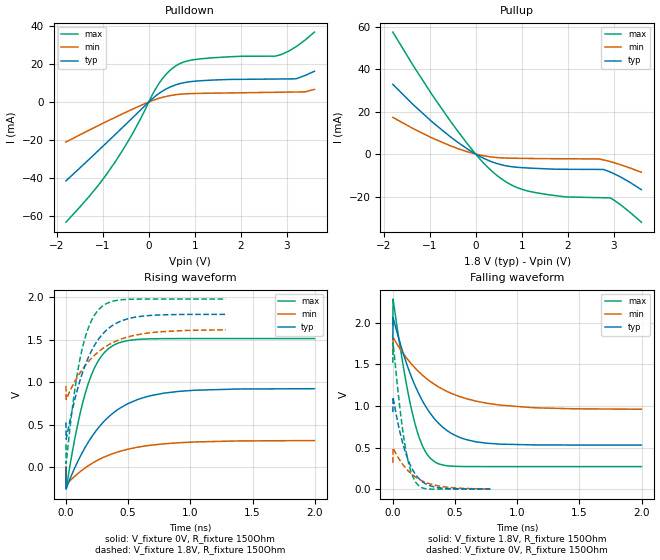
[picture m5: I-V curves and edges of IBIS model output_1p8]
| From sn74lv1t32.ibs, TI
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|   output_1p8 Model
[Model]   output_1p8
Model_type   Output
Polarity   Inverting
Vmeas = 0.9
Vref = 0
Cref = 30pF
Rref = 500
|   typ   min   max
|   (nom PVT)   (fast PVT)   (slow PVT)
C_comp   1.625e-12   1.538e-12   1.747e-12
| Where nom  PVT is Nominal Process, 1.8V, 40C
|   Fast PVT is Strong Process,  1.98V, -40C
|   Slow PVT is Weak Process,   1.62V, 140C
[Voltage Range]   1.8   1.62   1.98
|Junction Temperature
[Temperature Range]   40   140   -40
[Pullup Reference]   1.8   1.62   1.98
[Pulldown Reference]   0   0   0
[Power Clamp Reference]   1.8   1.62   1.98
[GND Clamp Reference]   0   0   0
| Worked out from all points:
|   slope of the pulldown table from 0 to 0.27 V, typ, clamps not added: 51.4 ohm
|   slope of the pullup table from 0 to 0.27 V, typ, clamps not added: 91.8 ohm
|   falling waveform, V_fixture 1.8V, R_fixture 150Ohm: 20-80 % time 271ps typ, 422ps min, 147ps max; typ from 1.8 V to 0.529 V
|   rising waveform, V_fixture 0V, R_fixture 150Ohm: 20-80 % time 351ps typ, 413ps min, 178ps max; typ from 0 V to 0.926 V
|   rising waveform, V_fixture 1.8V, R_fixture 150Ohm: 20-80 % time 213ps typ, 300ps min, 135ps max; typ from 0.529 V to 1.8 V
|   falling waveform, V_fixture 0V, R_fixture 150Ohm: 20-80 % time 129ps typ, 192ps min, 89.2ps max; typ from 0.926 V to 0.001 V
[Pulldown]
|   Voltage   I(typ)   I(min)   I(max)
-1.8V     -41.38mA   -20.97mA   -63.01mA
-1.282V   -29.71mA   -14.59mA   -49.12mA
-907.4mV  -21.14mA   -10.11mA   -37.57mA
-346.7mV  -8.144mA   -3.699mA   -16.34mA
146.3mV   3.113mA    1.347mA    6.829mA
308.7mV   5.851mA    2.524mA    12.6mA
496.8mV   8.174mA    3.493mA    17.32mA
684.9mV   9.69mA     4.077mA    20.23mA
996.1mV   10.89mA    4.456mA    22.24mA
2.832V    12.05mA    5.11mA     24.55mA
3.196V    12.13mA    5.233mA    28.93mA
3.6V      16.12mA    6.605mA    36.64mA
[Pullup]
|   Voltage   I(typ)   I(min)   I(max)
-1.8V     32.8mA     17.27mA    57.44mA
-964.4mV  15.51mA    7.761mA    28.52mA
-368.5mV  5.222mA    2.43mA     10.19mA
79.2mV    -961.8uA   -401.8uA   -2.013mA
528.5mV   -4.873mA   -1.755mA   -11.17mA
898.9mV   -6.226mA   -2.004mA   -15.78mA
1.331V    -6.775mA   -2.129mA   -18.29mA
1.978V    -7.178mA   -2.225mA   -20.21mA
2.776V    -7.258mA   -2.752mA   -20.58mA
2.926V    -8.494mA   -3.575mA   -20.65mA
3.17V     -11.06mA   -5.172mA   -24.25mA
3.6V      -16.77mA   -8.595mA   -32.09mA
[Ramp]
R_load = 150
|   typ   min   max
dV/dt_r   0.55539/3.51261e-10   0.189425/4.12478e-10   0.909405/1.77611e-10
dV/dt_f   0.762438/2.70787e-10   0.396415/4.2157e-10   1.02562/1.47306e-10
[Falling Waveform]
V_fixture = 1.8V
V_fixture_min = 1.62V
V_fixture_max = 1.98V
R_fixture = 150Ohm
|   Time   V(typ)   V(min)   V(max)
0s        1.8V       1.62V      1.98V
2ps       2.062V     1.822V     2.282V
110ps     1.51V      1.576V     1.255V
156ps     1.324V     1.492V     919.1mV
198ps     1.179V     1.425V     682.8mV
264ps     993.6mV    1.336V     445.1mV
344ps     828.8mV    1.249V     321.2mV
522ps     630.9mV    1.12V      273.1mV
754ps     551.8mV    1.032V     270.8mV
1.998ns   529.3mV    959.3mV    270.6mV
[Rising Waveform]
V_fixture = 0V
V_fixture_min = 0V
V_fixture_max = 0V
R_fixture = 150Ohm
|   Time   V(typ)   V(min)   V(max)
0s        377.5pV    9.214nV    426.7pV
2ps       -247.9mV   -204.4mV   -256.3mV
52ps      -67.54mV   -130.2mV   187.9mV
104ps     96.47mV    -62.83mV   570.1mV
204ps     352.7mV    41.84mV    1.084V
288ps     512.7mV    108.5mV    1.314V
388ps     649.1mV    167.6mV    1.441V
610ps     814.4mV    245.6mV    1.508V
902ps     893.2mV    289.4mV    1.515V
1.998ns   925.6mV    315.7mV    1.516V
[Rising Waveform]
V_fixture = 1.8V
V_fixture_min = 1.62V
V_fixture_max = 1.98V
R_fixture = 150Ohm
|   Time   V(typ)   V(min)   V(max)
0s        529.2mV    958.3mV    270.6mV
2ps       331.6mV    800.7mV    44.91mV
42ps      615.2mV    928mV      584.8mV
72ps      803mV      1.012V     921.9mV
138ps     1.135V     1.165V     1.439V
204ps     1.367V     1.282V     1.722V
290ps     1.56V      1.392V     1.893V
394ps     1.687V     1.48V      1.961V
562ps     1.769V     1.557V     1.979V
1.286ns   1.8V       1.618V     1.98V
[Falling Waveform]
V_fixture = 0V
V_fixture_min = 0V
V_fixture_max = 0V
R_fixture = 150Ohm
|   Time   V(typ)   V(min)   V(max)
0s        926mV      316.5mV    1.516V
2ps       1.104V     493.9mV    1.76V
52ps      719.6mV    357.6mV    1.037V
74ps      583.8mV    308.7mV    769.3mV
98ps      458.1mV    262.3mV    527.3mV
138ps     297mV      198.8mV    247.4mV
192ps     157.3mV    135.6mV    66.82mV
258ps     69.23mV    84.64mV    6.244mV
350ps     21.68mV    43.64mV    155.8uV
784ps     1.016mV    1.906mV    40.01uV
